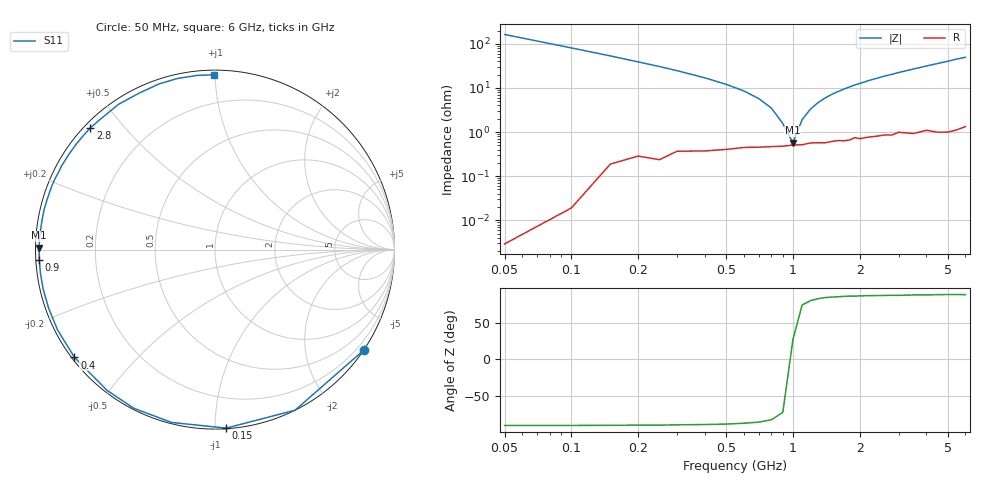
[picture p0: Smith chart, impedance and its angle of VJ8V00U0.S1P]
! Infineon Technologies  Discrete & RF Semiconductors
! BB 914
! Si Tuning Diode in SOT23
! VR = 8 V
! S-Parameters:  July  1999
# GHz  S  MA  R  50
!  f  S11
! GHz  MAG  ANG
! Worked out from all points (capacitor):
!   34 points, 50 MHz to 6 GHz, reference 50 ohm
!   read as one part to ground: C = 19.5 pF near 50 MHz
!   lowest |Z| = 571 mohm at 1 GHz (marker M1)
!   series resonance near 985 MHz, so ESL is about 1.3 nH
!   S11 on the Smith chart (normalised r, x): 50 MHz: 0.00, -3.26; 150 MHz: 0.00, -1.06; 400 MHz: 0.01, -0.34; 900 MHz: 0.01, -0.03; 2.8 GHz: 0.02, +0.41; 6 GHz: 0.03, +0.99
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0.05  1 -34.1
0.1  0.9998 -63.5
0.15  0.9965 -86.4
0.2  0.9929 -104.1
0.25  0.9931 -117.1
0.3  0.9883 -127.5
0.4  0.9867 -142.5
0.5  0.9849 -152.9
0.6  0.9828 -160.6
0.7  0.9822 -166.9
0.8  0.9815 -172.1
0.9  0.9811 -176.6
1  0.9799 179.4
1.1  0.9796 175.8
1.3  0.9775 169.4
1.5  0.9763 163.7
1.6  0.9753 161.2
1.9  0.9721 153.8
2.2  0.9721 147.2
2.4  0.9713 143.2
2.6  0.9702 139.1
2.8  0.971 135.6
3.5  0.9717 123.5
4  0.969 115.7
4.5  0.9741 108.6
5  0.9761 102.3
5.5  0.9755 95.7
6  0.9736 90.4
